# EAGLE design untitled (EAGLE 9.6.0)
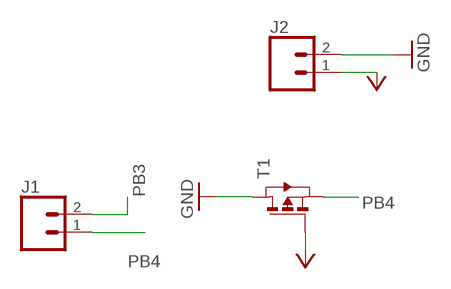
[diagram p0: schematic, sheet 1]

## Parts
J1  CONN_02  [1X02]
J2  CONN_02  [1X02]
T1  MOSFET_PSOT23  [SOT-23]

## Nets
GND: J2.2 T1.1(D)
PB3: J1.2
PB4: J1.1 T1.2(S)
VCC: J2.1 T1.3(G)

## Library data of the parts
J1 J2 = SparkFun-Connectors:CONN_02: Multi connection point. Often used as Generic Header-pin footprint for 0.1 inch spaced/style header connections
T1 = fab:MOSFET_P: MOS FET

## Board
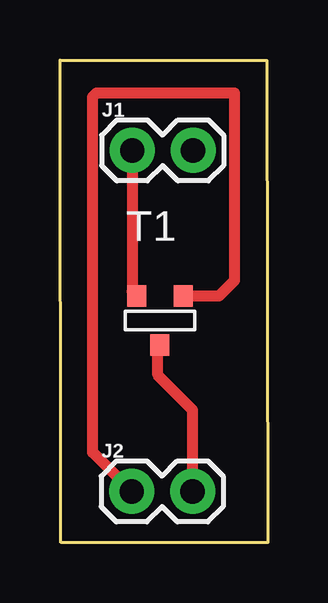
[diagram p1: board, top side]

Size 8.66 x 20.11 mm. Coordinates in mm from the lower left corner, seen from the top.
Outline: 0,20.11 8.62,20.09 8.66,0 0.04,0 0,20.11
Copper layers (1*16): Top 0.035mm / dielectric 1.5mm / Bottom 0.035mm
Design rules "default *": minimum track width 18mil, minimum drill 0.35mm, track to track 16mil, track to pad 16mil, pad to pad 16mil, via to via 6mil, smd to smd 16mil, copper to edge 40mil, drill to drill 6mil, minimum pad ring 10mil, minimum via ring 8mil, stop-mask expansion 4mil, vias tented up to drill 0mil, thermal gap 10mil

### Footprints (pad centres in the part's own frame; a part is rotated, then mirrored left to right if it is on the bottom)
1X02 = drill 1.016 pad 1.88: 1 0,0; 2 2.54,0
SOT-23 = smd 0.787 x 0.889: 1 0.025,-1.016; 2 -0.94,1.016; 3 0.991,1.016

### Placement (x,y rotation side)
J1  3.01,16.34 0 top
J2  2.99,2.13 0 top
T1  4.14,9.26 0 top

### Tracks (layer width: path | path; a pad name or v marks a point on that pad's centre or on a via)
GND
  Top 0.457: J2.2 5.53,5.53 4.08,6.98 4.08,8.15 T1.1
PB4
  Top 0.457: J1.1 3.01,10.46 T1.2
VCC
  Top 0.457: J2.1 1.36,3.76 1.36,18.57 1.53,18.74 7.27,18.74 7.27,10.92 6.62,10.27 T1.3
